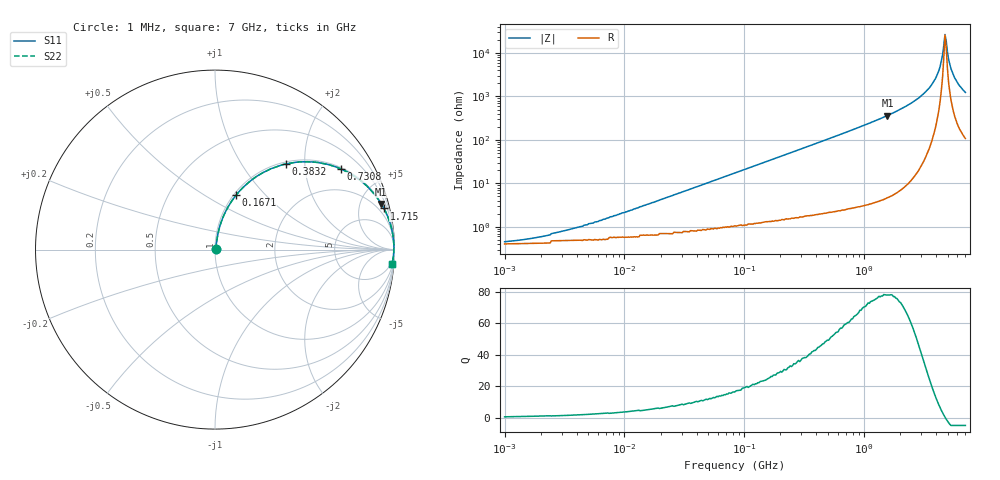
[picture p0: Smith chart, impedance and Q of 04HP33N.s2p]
# MHz S MA R 50
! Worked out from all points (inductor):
!   385 points, 1 MHz to 7 GHz, reference 50 ohm
!   read as one part in series: L = 33 nH near 8.341 MHz
!   highest Q = 78.2 at 1.564 GHz (marker M1), where L = 37 nH
!   self-resonance near 4.73 GHz
!   S11 on the Smith chart (normalised r, x): 1 MHz: 1.01, +0.00; 167.1 MHz: 1.03, +0.69; 383.2 MHz: 1.04, +1.60; 730.8 MHz: 1.05, +3.10; 1.715 GHz: 1.09, +8.18; 7 GHz: 3, -25
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1  0.004556 26.8  0.996 -0.1  0.996 -0.1  0.004556 26.8
4.374  0.01 61.0  0.995 -0.5  0.995 -0.5  0.01 61.0
19.575  0.041 78.3  0.992 -2.3  0.992 -2.3  0.041 78.3
85.617  0.173 76.6  0.975 -10.0  0.975 -10.0  0.173 76.6
167.089  0.324 68.9  0.934 -18.9  0.934 -18.9  0.324 68.9
365.931  0.6 51.8  0.786 -36.9  0.786 -36.9  0.6 51.8
383.2  0.618 50.5  0.772 -38.1  0.772 -38.1  0.618 50.5
730.797  0.834 32.5  0.538 -56.5  0.538 -56.5  0.834 32.5
1563.994  0.961 15.3  0.264 -73.9  0.264 -73.9  0.961 15.3
1637.803  0.965 14.5  0.25 -74.8  0.25 -74.8  0.965 14.5
1715.095  0.969 13.7  0.237 -75.6  0.237 -75.6  0.969 13.7
2848.264  0.992 6.2  0.108 -82.6  0.108 -82.6  0.992 6.2
3670.509  0.996 3.0  0.053 -84.1  0.053 -84.1  0.996 3.0
4025.125  0.997 1.9  0.034 -83.1  0.034 -83.1  0.997 1.9
4313.395  0.997 1.1  0.02 -79.7  0.02 -79.7  0.997 1.1
4516.955  0.997 0.6  0.011 -71.3  0.011 -71.3  0.997 0.6
4730.122  0.996 0.1  0.003739 -15.4  0.003739 -15.4  0.996 0.1
4840.449  0.996 -0.2  0.005223 44.2  0.005223 44.2  0.996 -0.2
5068.882  0.996 -0.7  0.014 72.1  0.014 72.1  0.996 -0.7
5308.095  0.995 -1.3  0.023 77.8  0.023 77.8  0.995 -1.3
5956.691  0.994 -2.6  0.046 80.9  0.046 80.9  0.994 -2.6
7000  0.99 -4.6  0.08 80.4  0.08 80.4  0.99 -4.6
